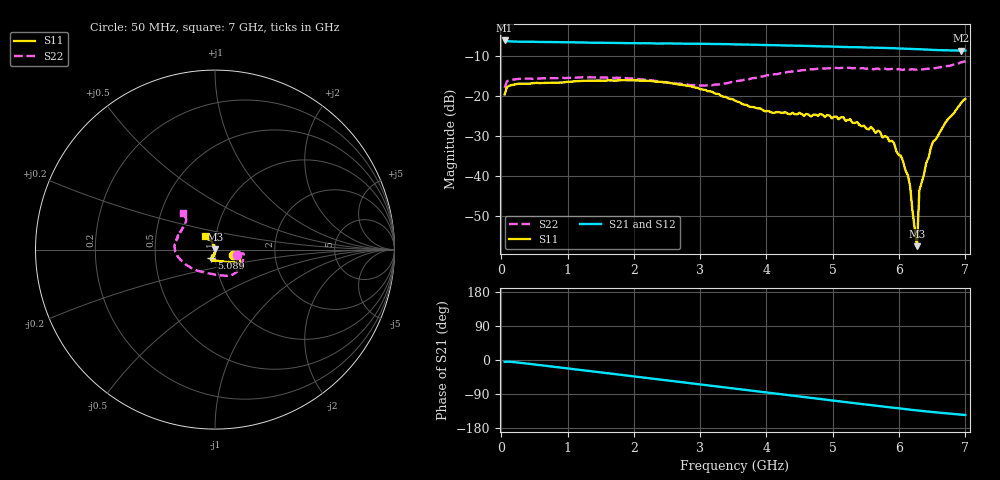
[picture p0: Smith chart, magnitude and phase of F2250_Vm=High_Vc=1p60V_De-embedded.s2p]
! Integrated Device Technology
! Corporate Headquarters
! 6024 Silver Creek Valley Road
! San Jose, CA 95138  USA
! Phone:  1-408-284-8200
! Toll Free:  1-800-223-1366
! Webpage:  http://www.idt.com/
! Timing and RF Division
! 515 Groton Road, Suite 102
! Westford, MA 01886-6024
! Device:  F2250
! Description: Voltage Variable RF Attenuator
! Frequency:  50.0 -  6000.00 MHz
! Package:  3x3 mm Thin QFN Plastic Package: 16 pin
! Ports:  2 RF, 3 DC
!  Pin  1  = GND
!  Pin  2  = NC
!  Pin  3  = RF1  = Port 1
!  Pin  4  = NC
!  Pin  5  = GND
!  Pin  6  = GND
!  Pin  7  = GND
!  Pin  8  = GND
!  Pin  9  = NC
!  Pin 10  = RF2  = Port 2
!  Pin 11  = NC
!  Pin 12  = GND
!  Pin 13  = GND
!  Pin 14  = VCNTRL
!  Pin 15  = VDD
!  Pin 16  = VMODE
! Vcntrl:  1.600 Volts
! Vmode:  +3.300 Volts
! Vdd:  +3.30  Volts
! Current:  1.328 mA
! Data:  The device was measured on a the F2250 evaluation board which has
!  individual transmission lines to the RF pins.  Data was collected
!  using a calibrated network analyzer.  The evaluation board was
!  de-embedded using a TRL calibration technique.
!  The reference plane is the edge of the package pin.
! Misc:  SN 10
!  Action Tracker AT0258
! Date Measured:  2014-11-26
! Date:  2015-10-15  MJV
! Note:
!  Integrated Device Technology supplies this data as a sample of measured
!  data at the package pin for this product.  Your particular data for this
!  product may vary.
!  Data was taken at 25 degrees C.
!  Integrated Device Technology reserves the right to change this data at anytime.
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# GHz S dB R 50
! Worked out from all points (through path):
!   201 points, 50 MHz to 7 GHz, reference 50 ohm
!   highest |S21| = -6.04 dB at 50 MHz (marker M1); lowest = -8.6 dB at 6.931 GHz (marker M2)
!   group delay of S21, straight-line fit = 58.2 ps
!   lowest |S11| = -57.4 dB at 6.27 GHz (marker M3), VSWR 1.00, Z = 50.1 + j0.113 ohm
!   |S11| at or under -10 dB: start of sweep to end of sweep
!   |S22| runs from -17.9 to -11.2 dB; largest |S21 - S12| = 0.0035
!   S11 on the Smith chart (normalised r, x): 50 MHz: 1.22, -0.08; 5.089 GHz: 0.96, -0.09; 7 GHz: 0.89, +0.14
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0.05  -19.54 -18.1  -6.04 -5.0  -6.04 -4.9  -17.88 -14.5
0.08475  -17.73 -9.3  -6.22 -4.3  -6.21 -4.3  -16.28 -8.7
0.2585  -16.84 -8.2  -6.35 -6.8  -6.34 -6.8  -15.66 -11.8
1.2315  -16.12 -25.2  -6.55 -27.2  -6.57 -27.2  -15.23 -42.8
2.37825  -16.36 -30.2  -6.80 -50.9  -6.79 -50.9  -16.18 -70.8
2.969  -17.95 -34.1  -6.86 -63.5  -6.87 -63.5  -17.33 -97.2
3.525  -21.07 -49.6  -7.02 -75.6  -7.00 -75.7  -16.31 -130.1
3.97675  -23.75 -74.3  -7.18 -85.4  -7.19 -85.4  -14.89 -151.9
4.7065  -24.59 -110.3  -7.44 -101.0  -7.47 -100.9  -13.25 -174.2
5.08875  -25.76 -112.9  -7.63 -109.0  -7.64 -109.0  -12.96 176.5
5.57525  -27.63 -108.4  -7.82 -118.9  -7.83 -119.0  -13.09 165.2
5.85325  -31.26 -100.2  -7.95 -124.7  -7.94 -124.8  -13.24 156.6
5.92275  -31.62 -98.4  -7.98 -126.1  -7.99 -126.1  -13.27 155.9
6.13125  -39.66 -91.1  -8.13 -130.2  -8.11 -130.4  -13.34 148.9
6.166  -42.45 -83.2  -8.14 -131.0  -8.13 -131.1  -13.32 147.2
6.20075  -48.36 -105.7  -8.17 -131.7  -8.17 -131.8  -13.20 146.5
6.27025  -57.44 57.1  -8.22 -133.0  -8.21 -133.1  -13.32 143.9
6.305  -43.56 104.2  -8.24 -133.7  -8.25 -133.8  -13.18 142.9
6.40925  -36.64 105.9  -8.33 -135.7  -8.34 -135.8  -13.11 139.2
6.5135  -31.28 107.5  -8.41 -137.4  -8.39 -137.6  -12.97 136.7
6.9305  -21.79 122.9  -8.57 -144.2  -8.56 -144.3  -11.52 131.6
7  -20.63 125.7  -8.56 -145.3  -8.57 -145.4  -11.23 131.2
